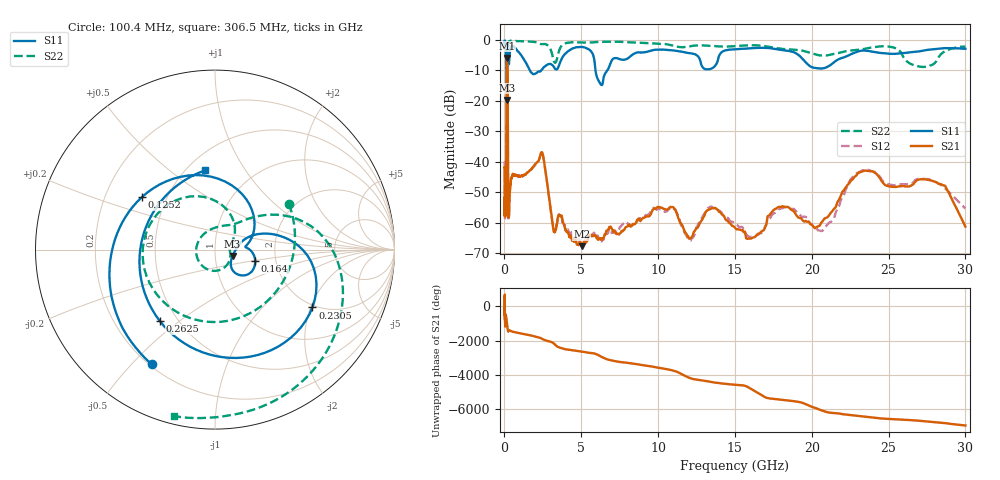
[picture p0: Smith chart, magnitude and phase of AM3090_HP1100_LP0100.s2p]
! Date/Time: Thu, Feb 28, 2019 2:06 PM
! Network Analyzer: Agilent Technologies E8364B Rev: A.07.50.67
! Sweep from 0.010 to 30.000 GHz, 1601 Points, Sweep Type: LOG
! Power Supply: 5.022 V, 0.002 A
# Hz S DB R 50
!freq MagS11 AngS11 MagS21 AngS21 MagS12 AngS12 MagS22 AngS22
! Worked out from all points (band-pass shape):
!   1601 points, 10 MHz to 30 GHz, reference 50 ohm
!   highest |S21| = -5.85 dB at 167.3 MHz (marker M1); lowest = -67.7 dB at 5.027 GHz (marker M2)
!   |S21| within 3 dB of the highest: 141 MHz to 201.5 MHz (60.49 MHz wide, 35.3 % of centre)
!   lowest |S11| = -19.6 dB at 194.4 MHz (marker M3), VSWR 1.23, Z = 60.7 - j4.3 ohm
!   |S11| at or under -10 dB: 136.3 MHz to 213.1 MHz (76.82 MHz wide, 44 % of centre); 1.649 GHz to 2.391 GHz (741.9 MHz wide, 36.7 % of centre); 5.926 GHz to 6.695 GHz (769.5 MHz wide, 12.2 % of centre)
!   |S22| runs from -21.8 to -0.1 dB; largest |S21 - S12| = 0.013
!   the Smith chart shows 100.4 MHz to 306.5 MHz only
!   S11 on the Smith chart (normalised r, x): 100.4 MHz: 0.21, -0.57; 125.2 MHz: 0.36, +0.28; 164 MHz: 1.56, -0.20; 230.5 MHz: 1.92, -2.06; 262.5 MHz: 0.40, -0.43; 306.5 MHz: 0.61, +0.68
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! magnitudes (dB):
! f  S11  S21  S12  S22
! 10 MHz  -0.2  -41.7  -40.2  -0.6
! 38.04 MHz  -0.4  -55.5  -56.8  -1.2
! 48.13 MHz  -0.6  -50.1  -46.1  -1.3
! 100.4 MHz  -2.7  -52.1  -53.9  -6.3
! 125.2 MHz  -6.0  -25.7  -25.7  -7.8
! 144.7 MHz  -14.7  -7.5  -7.5  -19.5
! 164 MHz  -12.7  -5.9  -5.9  -19.0
! 167.3 MHz  -12.4  -5.9  -5.8  -18.6
! 194.4 MHz  -19.6  -7.3  -7.3  -18.1
! 211.7 MHz  -10.8  -14.8  -14.8  -10.6
! 230.5 MHz  -4.0  -41.9  -42.3  -2.6
! 262.5 MHz  -6.0  -57.1  -57.0  -0.8
! 306.5 MHz  -7.0  -54.9  -57.6  -0.4
! 550.5 MHz  -2.0  -44.0  -44.3  -0.2
! 2.084 GHz  -10.8  -40.3  -40.3  -0.8
! 3.236 GHz  -9.0  -63.0  -62.4  -7.2
! 5.027 GHz  -2.3  -67.7  -66.7  -0.8
! 6.202 GHz  -14.0  -65.1  -65.2  -0.6
! 7.926 GHz  -6.3  -61.3  -59.8  -0.7
! 20.61 GHz  -9.4  -60.0  -62.7  -5.1
! 23.48 GHz  -3.5  -42.8  -42.6  -2.9
! 30 GHz  -2.9  -61.2  -55.3  -2.2
